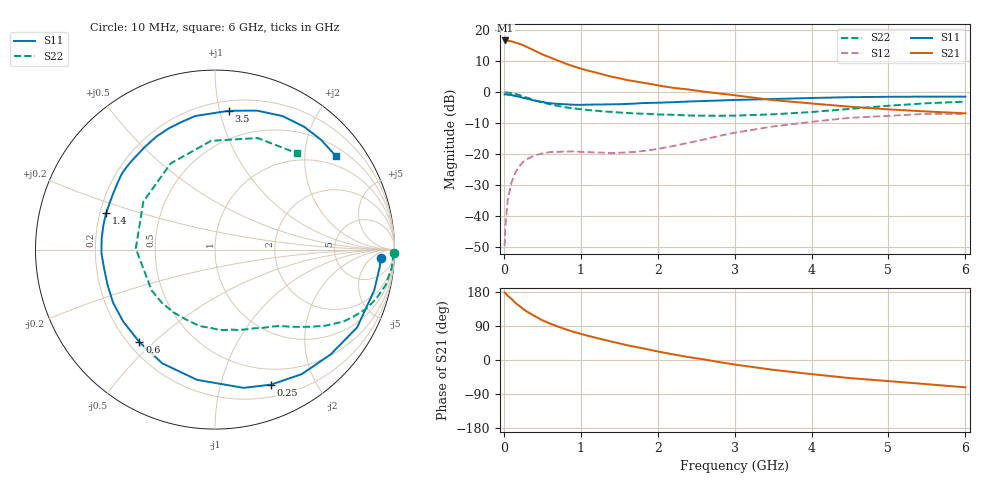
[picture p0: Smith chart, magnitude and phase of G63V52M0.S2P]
! SIEMENS Small Signal Semiconductors
! BFG193
! Si NPN RF Bipolar Junction Transistor in SOT223
! VCE = 3.5 V  IC = 2 mA
! Common Emitter S-Parameters:  August  1996
# GHz  S  MA  R  50
!  f  S11  S21  S12  S22
! GHz  MAG  ANG  MAG  ANG  MAG  ANG  MAG  ANG
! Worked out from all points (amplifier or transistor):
!   36 points, 10 MHz to 6 GHz, reference 50 ohm
!   highest |S21| = 16.7 dB at 20 MHz (marker M1)
!   |S21| within 3 dB of that: start of sweep to 376 MHz
!   unconditionally stable (mu >= 1): 1.362 GHz to 2.559 GHz
!   at 250 MHz: K = 0.18, MSG = 18.8 dB, |S12| = -22.5 dB
!   at 1.4 GHz: K = 1.04, MAG = 11.2 dB, |S12| = -19.6 dB
!   at 6 GHz: K = 0.95, MSG = 0.1 dB, |S12| = -6.9 dB
!   S11 on the Smith chart (normalised r, x): 10 MHz: 18, -12; 250 MHz: 0.32, -1.45; 600 MHz: 0.24, -0.45; 1.4 GHz: 0.23, +0.15; 3.5 GHz: 0.27, +1.07; 6 GHz: 0.72, +2.75
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0.01  0.9251 -2.9  6.819 177.8  0.0033 90.5  0.9952 -1.2
0.02  0.9231 -6.0  6.849 176.8  0.0069 84.2  0.9932 -2.3
0.05  0.9157 -14.4  6.789 169.4  0.0181 81.1  0.9895 -6.0
0.1  0.9027 -28.7  6.626 161.1  0.0353 74.9  0.9715 -11.7
0.15  0.8696 -42.2  6.333 150.8  0.0508 66.3  0.9379 -17.1
0.25  0.8145 -67.4  5.75 134.9  0.0753 53.7  0.8573 -25.8
0.3  0.7868 -78.3  5.377 127.7  0.0836 48.9  0.8208 -29.2
0.4  0.7326 -97.8  4.693 116.1  0.096 39.9  0.7454 -34.7
0.5  0.6986 -114.8  4.085 104.9  0.1033 33.0  0.6858 -38.8
0.6  0.6656 -129.3  3.648 96.2  0.1085 28.1  0.6399 -42.3
0.7  0.6499 -141.8  3.256 88.4  0.1096 24.4  0.6041 -45.4
0.8  0.6406 -152.3  2.908 81.2  0.1105 21.4  0.5724 -48.2
0.9  0.6302 -161.8  2.637 74.8  0.1114 19.8  0.5514 -50.6
1.1  0.6329 -178.3  2.225 63.6  0.1083 18.0  0.5173 -57.0
1.4  0.6397 161.6  1.781 48.6  0.1045 19.5  0.4821 -66.8
1.6  0.6487 150.5  1.575 39.0  0.1072 23.1  0.4649 -74.4
2.2  0.6919 124.8  1.179 14.9  0.136 32.7  0.4344 -101.2
2.8  0.7364 104.1  0.957 -5.5  0.1982 31.0  0.4187 -135.1
3.5  0.7775 84.3  0.748 -25.9  0.281 16.8  0.4413 179.2
4.5  0.8338 63.2  0.585 -47.8  0.3874 -7.6  0.5401 117.2
5.5  0.8505 46.0  0.49 -63.8  0.4489 -36.5  0.6654 69.1
6  0.8518 37.8  0.458 -72.2  0.4503 -51.9  0.7058 49.4
